DATA_BLOCK DB53
TITLE =

AUTHOR:INA
FAMILY:MotionIn
NAME:nb
VERSION:00.00


    FB53


BEGIN
       Read:=FALSE
       NodeID:=B#16#00
       Done:=FALSE
       Err:=FALSE
       ErrNo:=L#0
       PositionIs:=L#0
       xEdgeMerker:=FALSE
       xEdgeFlag:=FALSE
       xBusy:=FALSE
       xStep:=0

END_DATA_BLOCK
